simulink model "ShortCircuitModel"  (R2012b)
settings: Solver=ode45  StartTime=0.0  StopTime=120  RelTol=1e-3
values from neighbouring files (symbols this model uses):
  A = 50e-4    (= 0.005)    [SCmodel.m]
  Cp = 800    [SCmodel.m]
  h = 10    [SCmodel.m]
  m = 70e-3    (= 0.07)    [SCmodel.m]
  Q = 2*3600    (= 7200)    [SCmodel.m]    (also in PowerInputValidationTest.m; SimulationScript.m)
  Rshort = 0.5    [SCmodel.m]
  SOC = [0 0.1 0.2 0.3 0.4 0.5 0.6 0.7 0.8 0.9 1]    [SCmodel.m]    (also in PowerInputValidationTest.m; SimulationScript.m; int_series.m = 1:1:101)
  SOC_0 = 0.5    [SCmodel.m]    (also in PowerInputValidationTest.m; SimulationScript.m)
  T_inf = 20    [SCmodel.m]
  V = [2.25 3.2 3.25 3.25 3.3 3.3 3.3 3.35 3.35 3.35 3.75]    [SCmodel.m]    (also in PowerInputValidationTest.m; SimulationScript.m; int_series.m = [2.000; 2.760; 2.885; 2.963; 3.020; 3.066; 3.103; 3.136; 3.1)
undefined symbols (not defined in the file or in its folder): InitialSOC

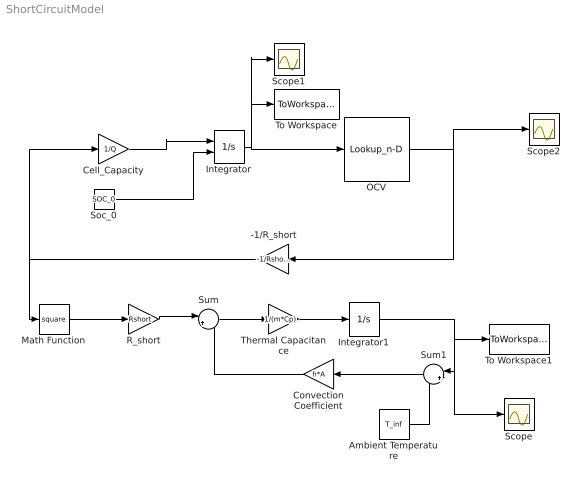
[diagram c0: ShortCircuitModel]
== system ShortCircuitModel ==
  -1/R_short : Gain  Gain=-1/Rshort
  Ambient Temperature : Constant  Value=T_inf
  Cell_Capacity : Gain  Gain=1/Q
  Convection Coefficient : Gain  Gain=h*A
  Integrator : Integrator  InitialConditionSource=external  InitialCondition=InitialSOC
  Integrator1 : Integrator  InitialCondition=T_inf  ZeroCross=off
  Math Function : Math  Operator=square
  OCV : Lookup_n-D  NumberOfTableDimensions=1  BreakpointsForDimension1=SOC  Table=V  RndMeth=Simplest
  R_short : Gain  Gain=Rshort
  Scope : Scope
  Scope1 : Scope
  Scope2 : Scope
  Soc_0 : Constant  Value=SOC_0
  Sum : Sum  Inputs=|+-
  Sum1 : Sum  Inputs=|+-
  Thermal Capacitance : Gain  Gain=1/(m*Cp)
  To Workspace : ToWorkspace  VariableName=stateofcharge  SampleTime=-1  SaveFormat=Structure With Time
  To Workspace1 : ToWorkspace  VariableName=Temp  SampleTime=-1  SaveFormat=Structure With Time
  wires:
  Integrator/1 -> OCV/1, Scope1/1, To Workspace/1
  Cell_Capacity/1 -> Integrator/1
  -1/R_short/1 -> Math Function/1, Cell_Capacity/1
  Soc_0/1 -> Integrator/2
  Convection Coefficient/1 -> Sum/2
  Sum/1 -> Thermal Capacitance/1
  Thermal Capacitance/1 -> Integrator1/1
  Math Function/1 -> R_short/1
  R_short/1 -> Sum/1
  Sum1/1 -> Convection Coefficient/1
  Integrator1/1 -> To Workspace1/1, Scope/1, Sum1/1
  Ambient Temperature/1 -> Sum1/2
  OCV/1 -> -1/R_short/1, Scope2/1
